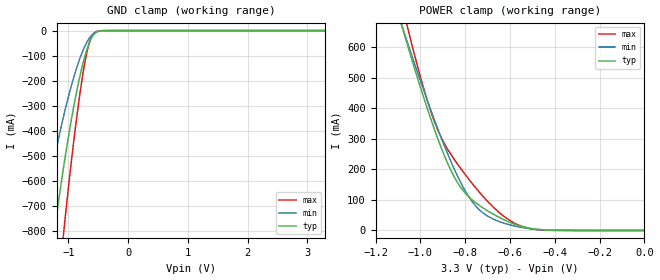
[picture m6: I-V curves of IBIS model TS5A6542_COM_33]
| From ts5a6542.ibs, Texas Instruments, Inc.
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[Model]   TS5A6542_COM_33
Model_type  Terminator
| variable   typ   min   max
C_comp   95.33pF   73.32pF   117.58pF
| C_tri-state   95.33pF   73.32pF   117.58pF
[Temperature Range]   40   100   -40
| Ambient temperature   25   85   -40
[Voltage range]   3.3   3   3.6
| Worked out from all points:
|   GND clamp passes 1 mA (typ) near -0.45 V on its own axis
|   POWER clamp passes 1 mA (typ) near -0.42 V on its own axis
[GND Clamp]
| TS5A6542_COM_33
|   Voltage   I(typ)   I(min)   I(max)
-3.3V     -5.832A    -4.179A    -7.751A
-1.465V   -1.238A    -801mA     -1.814A
-1.23V    -791.9mA   -502.8mA   -1.175A
-1.08V    -542.3mA   -340mA     -805mA
-900mV    -288.4mA   -177.5mA   -418.3mA
-755mV    -128.9mA   -78.09mA   -167.9mA
-705mV    -86.02mA   -52.29mA   -101.4mA
-655mV    -51.06mA   -31.87mA   -51.57mA
-600mV    -23.68mA   -16.05mA   -18.57mA
-545mV    -8.578mA   -6.744mA   -4.818mA
-315mV    -19.44uA   -37.7uA    -1.306uA
3.3V      6.409nA    70.16uA    3.516nA
[POWER Clamp]
| TS5A6542_COM_33
|   Voltage   I(typ)   I(min)   I(max)
-3.3V     8.004A     7.099A     9.576A
-1.09V    687.3mA    687.6mA    761.8mA
-1.07V    637.3mA    642.8mA    701.5mA
-1.05V    588mA      598.4mA    642.5mA
-990mV    445.9mA    469.3mA    477mA
-935mV    326mA      357.2mA    351.8mA
-870mV    206.3mA    236.4mA    255.9mA
-795mV    118.4mA    123.6mA    178.4mA
-720mV    73.53mA    57.17mA    111.3mA
-615mV    31.2mA     21.29mA    39.82mA
-515mV    7.753mA    6.195mA    6.549mA
-48.03fV  6.409nA    22.67nA    3.863nA
